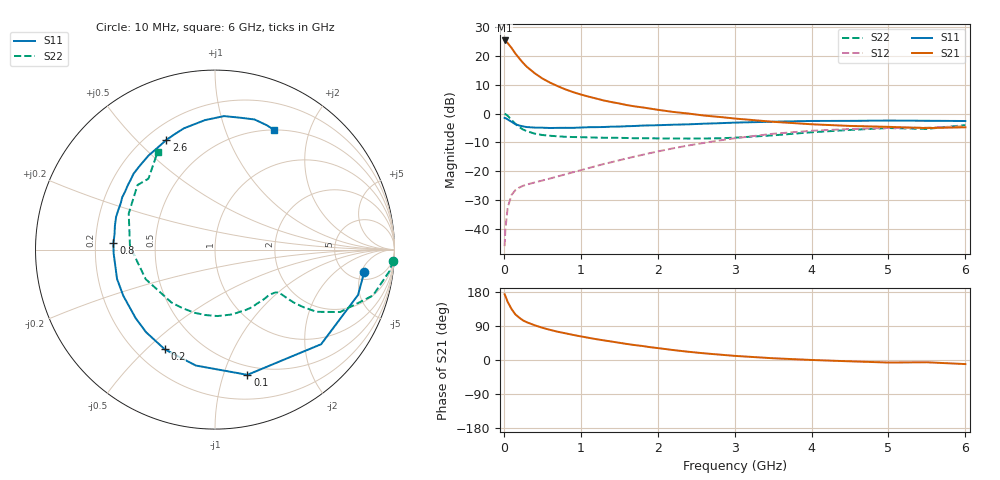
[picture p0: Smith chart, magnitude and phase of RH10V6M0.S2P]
! SIEMENS Small Signal Semiconductors
! BFR106
! Si NPN RF Bipolar Junction Transistor in SOT23
! VCE = 10 V  IC = 6 mA
! Common Emitter S-Parameters:  August  1996
# GHz  S  MA  R  50
!  f  S11  S21  S12  S22
! GHz  MAG  ANG  MAG  ANG  MAG  ANG  MAG  ANG
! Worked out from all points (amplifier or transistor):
!   36 points, 10 MHz to 6 GHz, reference 50 ohm
!   highest |S21| = 25.4 dB at 10 MHz (marker M1)
!   |S21| within 3 dB of that: start of sweep to 110.5 MHz
!   unconditionally stable (mu >= 1): 583.5 MHz to 1.838 GHz; 5.136 GHz to end of sweep
!   at 250 MHz: K = 0.55, MSG = 21.3 dB, |S12| = -25.1 dB
!   at 1.4 GHz: K = 1.12, MAG = 8.4 dB, |S12| = -16.9 dB
!   at 6 GHz: K = 1.01, MAG = -0.9 dB, |S12| = -4.4 dB
!   S11 on the Smith chart (normalised r, x): 10 MHz: 6.56, -5.68; 100 MHz: 0.41, -1.20; 200 MHz: 0.31, -0.57; 800 MHz: 0.28, +0.03; 2.6 GHz: 0.28, +0.61; 6 GHz: 0.50, +1.48
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0.01  0.8406 -8.7  18.61 173.6  0.005 89.8  0.9934 -3.6
0.02  0.836 -17.6  18.3 168.9  0.0097 82.5  0.98 -7.0
0.05  0.7923 -41.7  16.78 153.2  0.0234 69.7  0.9164 -16.2
0.1  0.7207 -75.5  13.81 134.5  0.0387 55.9  0.7793 -26.5
0.15  0.6547 -99.4  11.03 120.4  0.047 47.1  0.6636 -31.5
0.2  0.6223 -116.7  9.097 111.7  0.052 44.2  0.5865 -33.1
0.25  0.5994 -129.9  7.59 104.4  0.0559 42.4  0.5283 -33.9
0.3  0.584 -139.3  6.481 99.5  0.0587 42.8  0.4944 -34.0
0.4  0.572 -153.4  5.033 91.7  0.0638 43.8  0.4497 -33.9
0.5  0.5697 -163.3  4.077 85.1  0.0689 46.7  0.4252 -34.1
0.6  0.5626 -171.5  3.452 79.6  0.0747 49.4  0.4124 -35.4
0.8  0.5672 176.4  2.634 70.5  0.0882 54.9  0.3961 -39.1
1.1  0.5804 161.7  1.974 58.6  0.1132 60.9  0.3867 -46.8
1.3  0.5851 153.9  1.689 51.8  0.1335 63.2  0.3812 -52.7
1.6  0.6042 143.4  1.405 42.3  0.167 64.8  0.3773 -63.3
2.2  0.6416 125.3  1.07 26.3  0.2496 62.2  0.3705 -87.9
2.6  0.6683 114.0  0.926 17.7  0.3102 57.3  0.37 -107.9
3.5  0.7237 94.4  0.721 4.6  0.4467 42.0  0.4197 -156.9
4.5  0.7482 79.1  0.611 -3.5  0.5403 22.2  0.521 157.3
5  0.7577 73.1  0.589 -6.7  0.5638 13.6  0.5619 140.2
5.5  0.7506 67.4  0.561 -6.0  0.5693 9.1  0.5418 133.2
6  0.744 64.0  0.579 -10.8  0.606 0.8  0.6323 120.3
